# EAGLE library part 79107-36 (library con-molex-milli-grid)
RECEPTACAL
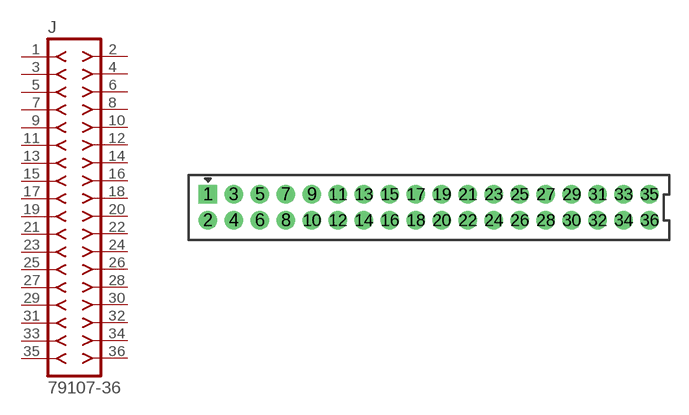
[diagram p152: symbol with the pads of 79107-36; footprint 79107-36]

Designator prefix J

## 79107-36  [79107-36]
1  1  pas
2  2  pas
3  3  pas
4  4  pas
5  5  pas
6  6  pas
7  7  pas
8  8  pas
9  9  pas
10  10  pas
11  11  pas
12  12  pas
13  13  pas
14  14  pas
15  15  pas
16  16  pas
17  17  pas
18  18  pas
19  19  pas
20  20  pas
21  21  pas
22  22  pas
23  23  pas
24  24  pas
25  25  pas
26  26  pas
27  27  pas
28  28  pas
29  29  pas
30  30  pas
31  31  pas
32  32  pas
33  33  pas
34  34  pas
35  35  pas
36  36  pas

## Footprint 79107-36 (pad centres in mm)
RECEPTACAL Dual Row, Vertical, Through-Hole
drill 0.914 square: 1 -17,1
drill 0.914: 2 -17,-1; 3 -15,1; 4 -15,-1; 5 -13,1; 6 -13,-1; 7 -11,1; 8 -11,-1; 9 -9,1; 10 -9,-1; 11 -7,1; 12 -7,-1; 13 -5,1; 14 -5,-1; 15 -3,1; 16 -3,-1; 17 -1,1; 18 -1,-1; 19 1,1; 20 1,-1; 21 3,1; 22 3,-1; 23 5,1; 24 5,-1; 25 7,1; 26 7,-1; 27 9,1; 28 9,-1; 29 11,1; 30 11,-1; 31 13,1; 32 13,-1; 33 15,1; 34 15,-1; 35 17,1; 36 17,-1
